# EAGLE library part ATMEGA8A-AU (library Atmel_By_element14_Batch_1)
Programmable Flash
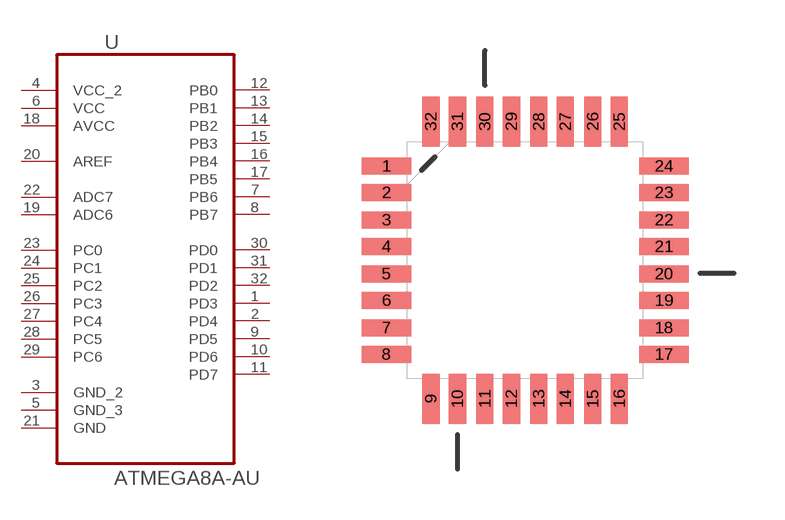
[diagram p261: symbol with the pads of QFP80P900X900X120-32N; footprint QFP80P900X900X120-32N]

Designator prefix U

## ATMEGA8A-AU (MPN: ATMEGA8A-AU; OC_FARNELL: 1748532; OC_NEWARK: 26R5638; PACKAGE: TQFP-32; SUPPLIER: Atmel)  [QFP80P900X900X120-32N]
1  PD3
2  PD4
3  GND_2  pas
4  VCC_2  pwr
5  GND_3  pas
6  VCC  pwr
7  PB6
8  PB7  pas
9  PD5  pas
10  PD6  pas
11  PD7  pas
12  PB0  pas
13  PB1  pas
14  PB2  pas
15  PB3  pas
16  PB4  pas
17  PB5  pas
18  AVCC  pwr
19  ADC6  in
20  AREF  in
21  GND  pas
22  ADC7  in
23  PC0
24  PC1
25  PC2
26  PC3
27  PC4
28  PC5
29  PC6
30  PD0
31  PD1
32  PD2

## Footprint QFP80P900X900X120-32N (pad centres in mm)
smd 1.473 x 0.508: 1 -4.115,2.794; 2 -4.115,2.007; 3 -4.115,1.194; 4 -4.115,0.406; 5 -4.115,-0.406; 6 -4.115,-1.194; 7 -4.115,-2.007; 8 -4.115,-2.794; 17 4.115,-2.794; 18 4.115,-2.007; 19 4.115,-1.194; 20 4.115,-0.406; 21 4.115,0.406; 22 4.115,1.194; 23 4.115,2.007; 24 4.115,2.794
smd 0.508 x 1.473: 9 -2.794,-4.115; 10 -2.007,-4.115; 11 -1.194,-4.115; 12 -0.406,-4.115; 13 0.406,-4.115; 14 1.194,-4.115; 15 2.007,-4.115; 16 2.794,-4.115; 25 2.794,4.115; 26 2.007,4.115; 27 1.194,4.115; 28 0.406,4.115; 29 -0.406,4.115; 30 -1.194,4.115; 31 -2.007,4.115; 32 -2.794,4.115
